| TEXAS INSTRUMENTS INCORPORATED
| Standard Linear and Logic Group
| IBIS Model of SN74ALVCH16245
| 16-BIT BUS TRANSCEIVER WITH 3-STATE OUTPUTS
| This file contains package information for the following:
|  TSSOP 48-pin (DGG) package as [Component] ALVCH16245_DGG
|  TVSOP 48-pin (DGV) package as [Component] ALVCH16245_DGV
|  SSOP 48-pin (DL) package as [Component] ALVCH16245_DL
|  VFBGA 48-pin (GQL) package as [Component] ALVCH16245_GQL
| This device can be powered at the following Vccs:
|  1.8 volt Vcc
|  2.5 volt Vcc
|  3.3 volt Vcc
| This file provides unique models under the [Model Selector] for each Vcc.
| For operation at a specific Vcc, select the appropriate model after each
| [Model Selector] keyword.
[IBIS Ver]   3.2
[Comment char]  |_char
[File Name]   sn74alvch16245.ibs
[File Rev]   1.1 | b_die
[Date]   March 21, 2002
[Source]   Data created from TI-SPICE simulations at TI-SLL.
[Notes]   The following is an IBIS list for the ALVCH16245.
   Please contact sllibis@ti.com with questions and
   comments concerning SLL IBIS models.
   This IBIS model is created from a BA (back annotated netlist
   - Due to presence of BUS-HOLD at input, GND-CLAMP curves
   have non-monotonic warnings.
[Disclaimer] Property of Texas Instruments Incorporated.  Unauthorized
   reproduction and/or distribution is strictly prohibited.
   This product is protected under copyright law.
   Created  2002, (C) Copyright  2002, Texas Instruments
   Incorporated, All Rights Reserved
   UNLESS THERE IS A SIGNED, WRITTEN AGREEMENT TO THE
   CONTRARY, TEXAS INSTRUMENTS (TI) IS PROVIDING THE IBIS
   MODELS  AND WITHOUT ANY WARRANTY, EXPRESSED OR
   IMPLIED.  TI assumes no liability for:
   1) the accuracy of the IBIS models provided to your
   company;
   2) the proper functioning of these IBIS Models in your
   design or for any resulting applications; or
   3) infringement of patents, copyrights or intellectual
   property rights resulting from your use of these IBIS
   models.
   TI provides IBIS Models as a service to our customers.
   You and your company shall not distribute, sell or give
   these models to anyone else without prior written
   permission from TI.
   TI reserves the right to make changes to our products or
   to discontinue any semiconductor product or service
   without notice, and advises our customers to obtain the
   latest version of relevant information to verify, before
   placing orders, that the information being relied on is
   current.
   Please be aware that your receipt and use of the IBIS
   information provided shall serve as acceptance of these
   terms and conditions.  If you do not accept these terms,
   you should return or destroy the IBIS models and any
   other accompanying information immediately.
| Component ALVCH16245_DGG 48-pin TSSOP
[Component]   ALVCH16245_DGG
[Manufacturer]   Texas Instruments, Inc.
[Package]
|   typ   min   max
R_pkg   4.400e-02   3.800e-02   5.100e-02
L_pkg   3.019e-09   2.486e-09   4.099e-09
C_pkg   5.070e-13   3.340e-13   8.090e-13
[Pin]   signal_name   model_name   R_pin   L_pin   C_pin
1   1DIR   ALVCH16245_DIR   4.100e-02   4.017e-09   7.590e-13
2   1B1   ALVCH16245_IO   4.200e-02   3.737e-09   7.920e-13
3   1B2   ALVCH16245_IO   4.200e-02   3.480e-09   6.610e-13
4   GND   GND   3.800e-02   3.131e-09   5.750e-13
5   1B3   ALVCH16245_IO   4.700e-02   3.122e-09   5.660e-13
6   1B4   ALVCH16245_IO   4.300e-02   2.948e-09   5.040e-13
7   VCC   POWER   4.500e-02   2.845e-09   3.970e-13
8   1B5   ALVCH16245_IO   4.900e-02   2.835e-09   3.940e-13
9   1B6   ALVCH16245_IO   4.800e-02   2.715e-09   3.780e-13
10   GND   GND   5.000e-02   2.664e-09   3.630e-13
11   1B7   ALVCH16245_IO   5.000e-02   2.585e-09   3.480e-13
12   1B8   ALVCH16245_IO   4.900e-02   2.550e-09   3.370e-13
13   2B1   ALVCH16245_IO   4.900e-02   2.541e-09   3.360e-13
14   2B2   ALVCH16245_IO   5.000e-02   2.574e-09   3.480e-13
15   GND   GND   4.900e-02   2.618e-09   3.590e-13
16   2B3   ALVCH16245_IO   4.600e-02   2.671e-09   3.750e-13
17   2B4   ALVCH16245_IO   4.500e-02   2.754e-09   3.890e-13
18   VCC   POWER   4.400e-02   2.823e-09   4.500e-13
19   2B5   ALVCH16245_IO   4.200e-02   2.968e-09   5.030e-13
20   2B6   ALVCH16245_IO   5.100e-02   3.108e-09   5.350e-13
21   GND   GND   4.200e-02   3.175e-09   5.870e-13
22   2B7   ALVCH16245_IO   4.100e-02   3.449e-09   6.780e-13
23   2B8   ALVCH16245_IO   4.400e-02   3.766e-09   8.040e-13
24   2DIR   ALVCH16245_DIR   4.300e-02   4.065e-09   7.610e-13
25   2OE   ALVCH16245_DIR   4.100e-02   3.994e-09   7.570e-13
26   2A8   ALVCH16245_IO   3.900e-02   3.649e-09   7.890e-13
27   2A7   ALVCH16245_IO   3.800e-02   3.362e-09   6.600e-13
28   GND   GND   3.800e-02   3.082e-09   5.740e-13
29   2A6   ALVCH16245_IO   4.400e-02   2.990e-09   5.220e-13
30   2A5   ALVCH16245_IO   4.100e-02   2.917e-09   4.950e-13
31   VCC   POWER   4.300e-02   2.820e-09   4.480e-13
32   2A4   ALVCH16245_IO   4.300e-02   2.699e-09   3.850e-13
33   2A3   ALVCH16245_IO   4.500e-02   2.628e-09   3.720e-13
34   GND   GND   4.600e-02   2.556e-09   3.560e-13
35   2A2   ALVCH16245_IO   4.600e-02   2.495e-09   3.440e-13
36   2A1   ALVCH16245_IO   4.700e-02   2.487e-09   3.340e-13
37   1A8   ALVCH16245_IO   4.700e-02   2.490e-09   3.350e-13
38   1A7   ALVCH16245_IO   4.600e-02   2.486e-09   3.430e-13
39   GND   GND   4.500e-02   2.566e-09   3.560e-13
40   1A6   ALVCH16245_IO   4.400e-02   2.639e-09   3.740e-13
41   1A5   ALVCH16245_IO   4.300e-02   2.701e-09   3.860e-13
42   VCC   POWER   4.300e-02   2.817e-09   4.500e-13
43   1A4   ALVCH16245_IO   4.100e-02   2.935e-09   5.010e-13
44   1A3   ALVCH16245_IO   4.700e-02   3.035e-09   5.290e-13
45   GND   GND   4.300e-02   3.171e-09   5.890e-13
46   1A2   ALVCH16245_IO   4.000e-02   3.415e-09   6.820e-13
47   1A1   ALVCH16245_IO   4.300e-02   3.741e-09   8.090e-13
48   1OE   ALVCH16245_DIR   4.400e-02   4.099e-09   7.640e-13
| Component ALVCH16245_DGV 48-pin TVSOP
[Component]   ALVCH16245_DGV
[Manufacturer]   Texas Instruments, Inc.
[Package]
|   typ   min   max
R_pkg   7.000e-02   4.900e-02   8.500e-02
L_pkg   3.013e-09   2.743e-09   3.408e-09
C_pkg   3.710e-13   2.940e-13   5.110e-13
[Pin]   signal_name   model_name   R_pin   L_pin   C_pin
1   1DIR   ALVCH16245_DIR   4.900e-02   3.393e-09   4.970e-13
2   1B1   ALVCH16245_IO   6.000e-02   3.250e-09   5.020e-13
3   1B2   ALVCH16245_IO   7.700e-02   3.310e-09   4.510e-13
4   GND   GND   8.500e-02   3.299e-09   4.040e-13
5   1B3   ALVCH16245_IO   8.300e-02   3.136e-09   3.600e-13
6   1B4   ALVCH16245_IO   7.700e-02   3.019e-09   3.630e-13
7   VCC   POWER   6.500e-02   2.882e-09   3.490e-13
8   1B5   ALVCH16245_IO   6.600e-02   2.829e-09   3.140e-13
9   1B6   ALVCH16245_IO   6.700e-02   2.796e-09   3.140e-13
10   GND   GND   6.900e-02   2.754e-09   3.080e-13
11   1B7   ALVCH16245_IO   7.000e-02   2.753e-09   3.010e-13
12   1B8   ALVCH16245_IO   7.100e-02   2.745e-09   2.940e-13
13   2B1   ALVCH16245_IO   7.000e-02   2.744e-09   2.940e-13
14   2B2   ALVCH16245_IO   7.000e-02   2.754e-09   3.010e-13
15   GND   GND   6.900e-02   2.754e-09   3.080e-13
16   2B3   ALVCH16245_IO   6.700e-02   2.796e-09   3.140e-13
17   2B4   ALVCH16245_IO   6.600e-02   2.829e-09   3.140e-13
18   VCC   POWER   6.500e-02   2.883e-09   3.500e-13
19   2B5   ALVCH16245_IO   7.500e-02   3.014e-09   3.630e-13
20   2B6   ALVCH16245_IO   8.000e-02   3.128e-09   3.580e-13
21   GND   GND   8.400e-02   3.295e-09   4.030e-13
22   2B7   ALVCH16245_IO   7.800e-02   3.311e-09   4.520e-13
23   2B8   ALVCH16245_IO   6.200e-02   3.259e-09   5.010e-13
24   2DIR   ALVCH16245_DIR   5.200e-02   3.404e-09   4.960e-13
25   2OE   ALVCH16245_DIR   5.300e-02   3.397e-09   5.050e-13
26   2A8   ALVCH16245_IO   6.200e-02   3.249e-09   5.110e-13
27   2A7   ALVCH16245_IO   7.700e-02   3.308e-09   4.530e-13
28   GND   GND   8.200e-02   3.289e-09   4.030e-13
29   2A6   ALVCH16245_IO   7.800e-02   3.121e-09   3.590e-13
30   2A5   ALVCH16245_IO   7.400e-02   3.010e-09   3.630e-13
31   VCC   POWER   6.500e-02   2.883e-09   3.490e-13
32   2A4   ALVCH16245_IO   6.700e-02   2.829e-09   3.140e-13
33   2A3   ALVCH16245_IO   6.700e-02   2.795e-09   3.140e-13
34   GND   GND   6.900e-02   2.753e-09   3.070e-13
35   2A2   ALVCH16245_IO   7.000e-02   2.753e-09   3.010e-13
36   2A1   ALVCH16245_IO   7.000e-02   2.743e-09   2.940e-13
37   1A8   ALVCH16245_IO   7.000e-02   2.743e-09   2.940e-13
38   1A7   ALVCH16245_IO   7.000e-02   2.753e-09   3.010e-13
39   GND   GND   6.900e-02   2.754e-09   3.070e-13
40   1A6   ALVCH16245_IO   6.800e-02   2.797e-09   3.140e-13
41   1A5   ALVCH16245_IO   6.700e-02   2.830e-09   3.140e-13
42   VCC   POWER   6.400e-02   2.880e-09   3.490e-13
43   1A4   ALVCH16245_IO   7.200e-02   3.004e-09   3.620e-13
44   1A3   ALVCH16245_IO   7.800e-02   3.121e-09   3.590e-13
45   GND   GND   8.400e-02   3.296e-09   4.030e-13
46   1A2   ALVCH16245_IO   7.700e-02   3.308e-09   4.510e-13
47   1A1   ALVCH16245_IO   6.200e-02   3.258e-09   4.990e-13
48   1OE   ALVCH16245_DIR   5.300e-02   3.408e-09   4.940e-13
| Component ALVCH16245_DL 48-pin SSOP
[Component]   ALVCH16245_DL
[Manufacturer]   Texas Instruments, Inc.
[Package]
|   typ   min   max
R_pkg   4.800e-02   3.800e-02   5.300e-02
L_pkg   6.046e-09   5.084e-09   7.968e-09
C_pkg   8.130e-13   5.690e-13   1.157e-12
[Pin]   signal_name   model_name   R_pin   L_pin   C_pin
1   1DIR   ALVCH16245_DIR   4.600e-02   7.968e-09   1.017e-12
2   1B1   ALVCH16245_IO   4.400e-02   7.299e-09   1.157e-12
3   1B2   ALVCH16245_IO   4.300e-02   6.765e-09   1.058e-12
4   GND   GND   4.100e-02   6.269e-09   9.330e-13
5   1B3   ALVCH16245_IO   3.800e-02   5.856e-09   8.290e-13
6   1B4   ALVCH16245_IO   4.600e-02   5.802e-09   7.900e-13
7   VCC   POWER   5.000e-02   5.656e-09   7.380e-13
8   1B5   ALVCH16245_IO   5.300e-02   5.500e-09   6.430e-13
9   1B6   ALVCH16245_IO   5.200e-02   5.304e-09   6.060e-13
10   GND   GND   5.300e-02   5.189e-09   5.830e-13
11   1B7   ALVCH16245_IO   5.100e-02   5.084e-09   5.690e-13
12   1B8   ALVCH16245_IO   5.300e-02   5.862e-09   8.330e-13
13   2B1   ALVCH16245_IO   5.300e-02   5.862e-09   8.330e-13
14   2B2   ALVCH16245_IO   5.100e-02   5.084e-09   5.690e-13
15   GND   GND   5.300e-02   5.189e-09   5.830e-13
16   2B3   ALVCH16245_IO   5.200e-02   5.304e-09   6.060e-13
17   2B4   ALVCH16245_IO   5.300e-02   5.500e-09   6.430e-13
18   VCC   POWER   5.000e-02   5.656e-09   7.380e-13
19   2B5   ALVCH16245_IO   4.600e-02   5.802e-09   7.900e-13
20   2B6   ALVCH16245_IO   3.800e-02   5.856e-09   8.290e-13
21   GND   GND   4.100e-02   6.269e-09   9.330e-13
22   2B7   ALVCH16245_IO   4.300e-02   6.765e-09   1.058e-12
23   2B8   ALVCH16245_IO   4.400e-02   7.299e-09   1.157e-12
24   2DIR   ALVCH16245_DIR   4.600e-02   7.968e-09   1.017e-12
25   2OE   ALVCH16245_DIR   4.600e-02   7.968e-09   1.017e-12
26   2A8   ALVCH16245_IO   4.400e-02   7.299e-09   1.157e-12
27   2A7   ALVCH16245_IO   4.300e-02   6.765e-09   1.058e-12
28   GND   GND   4.100e-02   6.269e-09   9.330e-13
29   2A6   ALVCH16245_IO   3.800e-02   5.856e-09   8.290e-13
30   2A5   ALVCH16245_IO   4.600e-02   5.802e-09   7.900e-13
31   VCC   POWER   5.000e-02   5.656e-09   7.380e-13
32   2A4   ALVCH16245_IO   5.300e-02   5.500e-09   6.430e-13
33   2A3   ALVCH16245_IO   5.200e-02   5.304e-09   6.060e-13
34   GND   GND   5.300e-02   5.189e-09   5.830e-13
35   2A2   ALVCH16245_IO   5.100e-02   5.084e-09   5.690e-13
36   2A1   ALVCH16245_IO   5.300e-02   5.862e-09   8.330e-13
37   1A8   ALVCH16245_IO   5.300e-02   5.862e-09   8.330e-13
38   1A7   ALVCH16245_IO   5.100e-02   5.084e-09   5.690e-13
39   GND   GND   5.300e-02   5.189e-09   5.830e-13
40   1A6   ALVCH16245_IO   5.200e-02   5.304e-09   6.060e-13
41   1A5   ALVCH16245_IO   5.300e-02   5.500e-09   6.430e-13
42   VCC   POWER   5.000e-02   5.656e-09   7.380e-13
43   1A4   ALVCH16245_IO   4.600e-02   5.802e-09   7.900e-13
44   1A3   ALVCH16245_IO   3.800e-02   5.856e-09   8.290e-13
45   GND   GND   4.100e-02   6.269e-09   9.330e-13
46   1A2   ALVCH16245_IO   4.300e-02   6.765e-09   1.058e-12
47   1A1   ALVCH16245_IO   4.400e-02   7.299e-09   1.157e-12
48   1OE   ALVCH16245_DIR   4.600e-02   7.967e-09   1.017e-12
| Component ALVCH16245_GQL 48-pin VFBGA
[Component]   ALVCH16245_GQL
[Manufacturer]   Texas Instruments, Inc.
[Package]
|   typ   min   max
R_pkg   7.900e-02   4.500e-02   9.400e-02
L_pkg   2.264e-09   1.398e-09   2.722e-09
C_pkg   3.060e-13   1.170e-13   4.040e-13
[Pin]   signal_name   model_name   R_pin   L_pin   C_pin
A1   1DIR   ALVCH16245_DIR  5.10E-02   1.53E-09   2.10E-13
B2   1B1   ALVCH16245_IO   7.30E-02   2.57E-09   3.12E-13
B1   1B2   ALVCH16245_IO   7.10E-02   1.84E-09   2.32E-13
B3   GND   GND   9.40E-02   2.72E-09   3.83E-13
C2   1B3   ALVCH16245_IO   8.90E-02   2.53E-09   3.50E-13
C1   1B4   ALVCH16245_IO   7.10E-02   1.83E-09   2.31E-13
C3   VCC   POWER   9.40E-02   2.72E-09   3.92E-13
D2   1B5   ALVCH16245_IO   9.00E-02   2.55E-09   3.52E-13
D1   1B6   ALVCH16245_IO   7.20E-02   1.85E-09   2.44E-13
D3   GND   GND   9.40E-02   2.72E-09   4.03E-13
E2   1B7   ALVCH16245_IO   8.90E-02   2.54E-09   3.51E-13
E1   1B8   ALVCH16245_IO   7.20E-02   1.85E-09   2.27E-13
F1   2B1   ALVCH16245_IO   7.20E-02   1.85E-09   2.27E-13
F2   2B2   ALVCH16245_IO   8.90E-02   2.54E-09   3.51E-13
G3   GND   GND   9.40E-02   2.72E-09   4.04E-13
G1   2B3   ALVCH16245_IO   7.20E-02   1.85E-09   2.44E-13
G2   2B4   ALVCH16245_IO   9.00E-02   2.55E-09   3.52E-13
H3   VCC   POWER   9.40E-02   2.72E-09   3.92E-13
H1   2B5   ALVCH16245_IO   7.00E-02   1.83E-09   2.31E-13
H2   2B6   ALVCH16245_IO   8.80E-02   2.52E-09   3.50E-13
J3   GND   GND   9.30E-02   2.71E-09   3.82E-13
J1   2B7   ALVCH16245_IO   7.10E-02   1.85E-09   2.33E-13
J2   2B8   ALVCH16245_IO   5.60E-02   2.61E-09   3.90E-13
K1   2DIR   ALVCH16245_DIR  4.50E-02   1.40E-09   1.17E-13
K6   2OE   ALVCH16245_DIR  4.50E-02   1.51E-09   1.93E-13
J5   2A8   ALVCH16245_IO   5.50E-02   2.49E-09   3.13E-13
J6   2A7   ALVCH16245_IO   7.00E-02   1.82E-09   2.30E-13
J4   GND   GND   9.30E-02   2.70E-09   3.82E-13
H5   2A6   ALVCH16245_IO   8.90E-02   2.53E-09   3.50E-13
H6   2A5   ALVCH16245_IO   7.10E-02   1.83E-09   2.30E-13
H4   VCC   POWER   9.40E-02   2.72E-09   3.91E-13
G5   2A4   ALVCH16245_IO   9.00E-02   2.55E-09   3.52E-13
G6   2A3   ALVCH16245_IO   7.20E-02   1.85E-09   2.44E-13
G4   GND   GND   9.40E-02   2.72E-09   4.04E-13
F5   2A2   ALVCH16245_IO   8.80E-02   2.51E-09   3.49E-13
F6   2A1   ALVCH16245_IO   7.20E-02   1.85E-09   2.27E-13
E6   1A8   ALVCH16245_IO   7.10E-02   1.85E-09   2.27E-13
E5   1A7   ALVCH16245_IO   8.90E-02   2.53E-09   3.50E-13
D4   GND   GND   9.40E-02   2.72E-09   4.03E-13
D6   1A6   ALVCH16245_IO   7.20E-02   1.85E-09   2.43E-13
D5   1A5   ALVCH16245_IO   8.90E-02   2.55E-09   3.52E-13
C4   VCC   POWER   9.40E-02   2.72E-09   3.91E-13
C6   1A4   ALVCH16245_IO   7.10E-02   1.83E-09   2.30E-13
C5   1A3   ALVCH16245_IO   8.90E-02   2.54E-09   3.50E-13
B4   GND   GND   9.30E-02   2.71E-09   3.82E-13
B6   1A2   ALVCH16245_IO   7.10E-02   1.83E-09   2.27E-13
B5   1A1   ALVCH16245_IO   7.30E-02   2.69E-09   3.80E-13
A6   1OE   ALVCH16245_DIR  5.10E-02   1.42E-09   1.33E-13
| Model ALVCH16245_DIR
[Model Selector]   ALVCH16245_DIR
ALVCH16245_DIR_18   1.8 volt Vcc
ALVCH16245_DIR_25   2.5 volt Vcc
ALVCH16245_DIR_33   3.3 volt Vcc
| Model ALVCH16245_IO
[Model Selector]   ALVCH16245_IO
ALVCH16245_IO_18   1.8 volt Vcc
ALVCH16245_IO_25   2.5 volt Vcc
ALVCH16245_IO_33   3.3 volt Vcc
| Models and submodels in the file (6): ALVCH16245_DIR_18 (Input), ALVCH16245_DIR_25 (Input), ALVCH16245_DIR_33 (Input), ALVCH16245_IO_18 (I/O), ALVCH16245_IO_25 (I/O), ALVCH16245_IO_33 (I/O)
